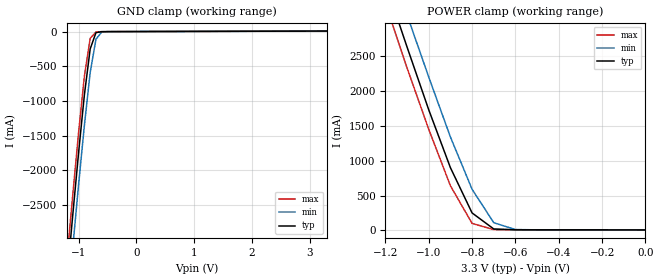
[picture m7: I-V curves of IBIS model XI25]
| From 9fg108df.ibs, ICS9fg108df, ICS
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|   Model XI25
[Model]   XI25
Model_type   Input
Polarity   Non-Inverting
Enable   Active-High
Vinl =   0.80V
Vinh =   2.00V
C_comp   5.50pF   5.00pF   6.00pF
[Temperature Range]   27.00   70.00   0.000
[Voltage Range]   3.30V   3.00V   3.70V
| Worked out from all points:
|   GND clamp passes 1 mA (typ) near -0.46 V on its own axis
[GND_clamp]
| voltage   I(typ)   I(min)   I(max)
-3.3V     -24.05A    -24.49A    -23.79A
-1.2V     -3.55A     -4.02A     -3.26A
-1.1V     -2.63A     -3.1A      -2.34A
-1V       -1.74A     -2.2A      -1.45A
-900mV    -910mA     -1.35A     -640mA
-800mV    -250mA     -590mA     -98.01mA
-700mV    -15.97mA   -110mA     -5.31mA
-600mV    -2.13mA    -7.05mA    -1.7mA
-500mV    -1.13mA    -1.39mA    -1.09mA
3.3V      6.89mA     6.89mA     6.89mA
[POWER_clamp]
| voltage   I(typ)   I(min)   I(max)
-3.3V     24.05A     24.48A     23.79A
-1.2V     3.55A      4.02A      3.26A
-1.1V     2.63A      3.09A      2.33A
-1V       1.73A      2.2A       1.45A
-900mV    900mA      1.34A      640mA
-800mV    250mA      590mA      100mA
-700mV    20.43mA    110mA      11.13mA
-600mV    8.42mA     12.3mA     9.01mA
0V        6.89mA     6.26mA     7.72mA
